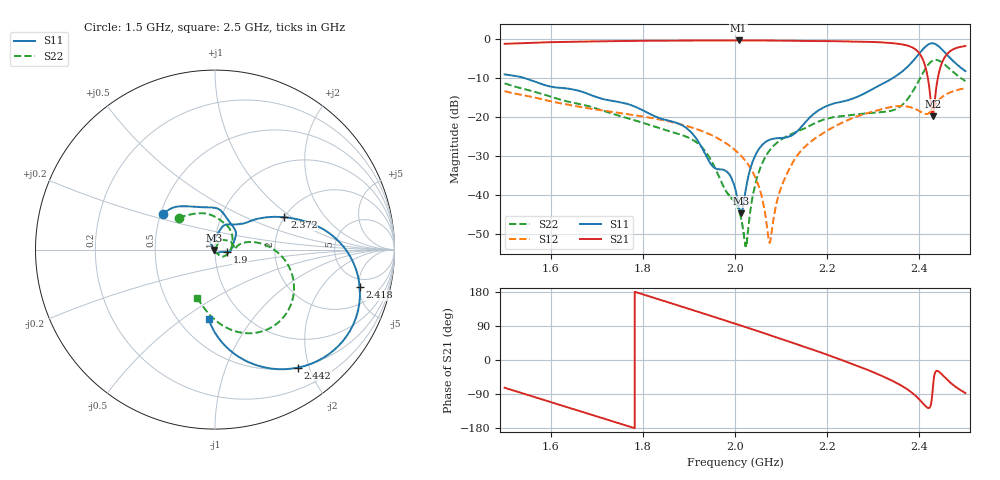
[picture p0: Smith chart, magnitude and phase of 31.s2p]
#  HZ  S  MA  R  50.00
! Rohde & Schwarz Vector Network Analyzer
! Rohde-Schwarz,ZNL6-2Port,1323001206101378,1.50.1.34-21.10.1.104
! Created: UTC 2/14/2025, 2:26:36 AM
! freq[Hz]  mag:S11  ang:S11  mag:S21  ang:S21  mag:S12  ang:S12  mag:S22  ang:S22
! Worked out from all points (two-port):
!   10001 points, 1.5 GHz to 2.5 GHz, reference 50 ohm
!   highest |S21| = -0.40 dB at 2.008 GHz (marker M1); lowest = -19.9 dB at 2.429 GHz (marker M2)
!   |S21| within 3 dB of the highest: start of sweep to 2.398 GHz; 2.464 GHz to end of sweep
!   lowest |S11| = -44.8 dB at 2.013 GHz (marker M3), VSWR 1.01, Z = 49.4 - j0.145 ohm
!   |S11| at or under -10 dB: 1.542 GHz to 2.343 GHz (801.4 MHz wide, 41.3 % of centre)
!   |S22| runs from -53.2 to -5.4 dB; largest |S21 - S12| = 1
!   S11 on the Smith chart (normalised r, x): 1.5 GHz: 0.52, +0.24; 1.9 GHz: 1.14, -0.03; 2.372 GHz: 2.00, +0.88; 2.418 GHz: 3.79, -5.15; 2.442 GHz: 0.49, -1.82; 2.5 GHz: 0.70, -0.63
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1.5e9  0.3505 145.2  0.8648 -73.2  0.2137 -106.3  0.2689 138.8
1.5827e9  0.2608 114.0  0.9031 -104.3  0.1673 -130.7  0.196 97.5
1.6667e9  0.2112 78.3  0.9229 -136.2  0.1332 -152.3  0.1443 57.5
1.8334e9  0.09763 9.4  0.9476 160.5  0.09319 159.5  0.07249 -21.2
1.8997e9  0.06798 -10.7  0.9518 135.1  0.075 135.8  0.0539 -46.6
2e9  0.01224 -104.5  0.9543 95.9  0.03764 95.3  0.008106 -130.9
2.0076e9  0.007651 -125.0  0.9545 92.9  0.03427 92.1  0.006529 -140.8
2.0132e9  0.005775 -165.3  0.9543 90.7  0.0317 89.8  0.005004 -149.8
2.0246e9  0.01295 134.7  0.9544 86.2  0.02634 85.1  0.002317 129.8
2.046e9  0.0338 125.0  0.9542 77.6  0.01575 77.6  0.01518 64.0
2.0755e9  0.0509 127.4  0.9523 65.6  0.002446 144.9  0.03746 65.6
2.1081e9  0.05402 114.0  0.9476 52.3  0.0162 -149.1  0.05464 68.6
2.1667e9  0.1041 77.1  0.9382 28.1  0.04921 -173.6  0.07941 41.2
2.2547e9  0.1704 55.0  0.9234 -10.4  0.09632 139.1  0.1058 11.8
2.3334e9  0.2922 35.9  0.8892 -50.2  0.1319 85.1  0.1176 4.7
2.3723e9  0.4263 25.0  0.8267 -76.0  0.136 42.9  0.1627 13.5
2.3957e9  0.605 11.3  0.699 -98.8  0.1229 0.6  0.2684 6.6
2.4176e9  0.8326 -14.5  0.3371 -125.9  0.109 -84.0  0.4528 -18.2
2.4291e9  0.8771 -34.0  0.1016 -77.5  0.1279 -148.0  0.5268 -38.0
2.4418e9  0.8038 -54.9  0.351 -30.2  0.1633 157.2  0.5276 -59.1
2.4609e9  0.6187 -76.9  0.645 -52.6  0.1985 108.1  0.4379 -82.0
2.5e9  0.3862 -95.3  0.8113 -87.2  0.2327 53.3  0.2881 -110.0
